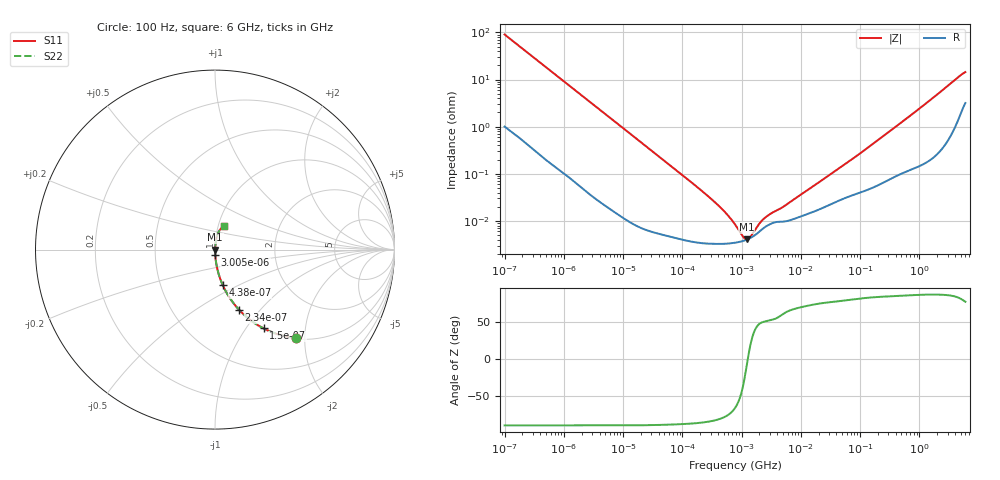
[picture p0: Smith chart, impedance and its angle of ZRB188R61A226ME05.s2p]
!Murata Part Number: ZRB188R61A226ME05
!These Parameters are Measured in Series Mode Connection
!Data Generated on Jun 10, 2025
!  o--ll--o
!Port1  Port2
!  o------o
!Operation Temp=25[degC], DC Bias Voltage=0[V]
!Freq. Start=100[Hz] Stop=6[GHz] 401[Steps]
# Hz S RI R 50
!Freq.(Hz) S11(Real) S11(Imag) S21(Real) S21(Imag) S12(Real) S12(Imag) S22(Real) S22(Imag)
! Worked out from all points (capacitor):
!   401 points, 100 Hz to 6 GHz, reference 50 ohm
!   read as one part in series: C = 17.6 uF near 109 Hz
!   lowest |Z| = 4.05 mohm at 1.212 MHz (marker M1)
!   series resonance near 1.273 MHz, so ESL is about 890 pH
!   S11 on the Smith chart (normalised r, x): 100 Hz: 1.02, -1.81; 150 Hz: 1.01, -1.21; 234 Hz: 1.01, -0.78; 438 Hz: 1.00, -0.42; 3.005 kHz: 1.00, -0.06; 6 GHz: 1.06, +0.28
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100  0.4501 -0.492  0.5499 0.492  0.5499 0.492  0.4501 -0.492
150  0.2707 -0.4387  0.7293 0.4387  0.7293 0.4387  0.2707 -0.4387
234  0.1339 -0.335  0.8661 0.335  0.8661 0.335  0.1339 -0.335
438  0.0436 -0.1989  0.9564 0.1989  0.9564 0.1989  0.0436 -0.1989
897  0.0114 -0.101  0.9886 0.101  0.9886 0.101  0.0114 -0.101
2008  0.00261 -0.0458  0.9974 0.0458  0.9974 0.0458  0.00261 -0.0458
3005  0.00128 -0.0307  0.9987 0.0307  0.9987 0.0307  0.00128 -0.0307
40335  5.86e-05 -0.00232  0.9999 0.00232  0.9999 0.00232  5.86e-05 -0.00232
241822  3.35e-05 -0.000379  1 0.000379  1 0.000379  3.35e-05 -0.000379
432798  3.26e-05 -0.000194  1 0.000194  1 0.000194  3.26e-05 -0.000194
677235  3.37e-05 -0.000101  1 0.000101  1 0.000101  3.37e-05 -0.000101
774597  3.45e-05 -7.72e-05  1 7.72e-05  1 7.72e-05  3.45e-05 -7.72e-05
1212075  3.99e-05 -7.2e-06  1 7.2e-06  1 7.2e-06  3.99e-05 -7.2e-06
2169299  6.5e-05 7.53e-05  0.9999 -7.53e-05  0.9999 -7.53e-05  6.5e-05 7.53e-05
3103719  8.67e-05 0.000113  0.9999 -0.000113  0.9999 -0.000113  8.67e-05 0.000113
5079039  9.68e-05 0.000175  0.9999 -0.000175  0.9999 -0.000175  9.68e-05 0.000175
1.555665e7  0.000153 0.000504  0.9998 -0.000504  0.9998 -0.000504  0.000153 0.000504
7.797396e7  0.000362 0.00213  0.9996 -0.00213  0.9996 -0.00213  0.000362 0.00213
3.124326e8  0.000817 0.00785  0.9992 -0.00785  0.9992 -0.00785  0.000817 0.00785
1.712697e9  0.00385 0.0408  0.9962 -0.0408  0.9962 -0.0408  0.00385 0.0408
4.586474e9  0.0262 0.1083  0.9738 -0.1083  0.9738 -0.1083  0.0262 0.1083
6e9  0.0484 0.1295  0.9516 -0.1295  0.9516 -0.1295  0.0484 0.1295
